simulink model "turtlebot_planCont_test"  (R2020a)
settings: Solver=FixedStepAuto  StartTime=0.0  StopTime=inf  RelTol=1e-3
PreLoadFcn:
  | addpath('../ros_fun')
model workspace (MAT data in the model file):
  SL_ROS_VariableLengthArrays_MaxSizes : object (value not decoded)
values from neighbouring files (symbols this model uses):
  desired_traj = zeros(size(pthObj.States,1),4)    [RRTstar_turtlebot.m]
undefined symbols (not defined in the file or in its folder): nav_msgs, Path, plan
libraries: robotlib x3

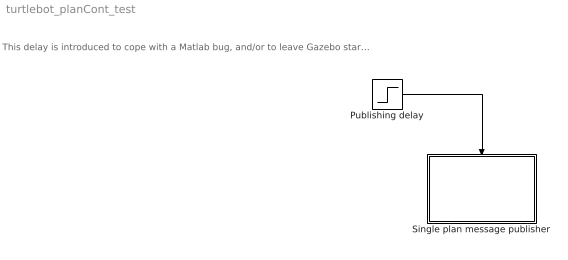
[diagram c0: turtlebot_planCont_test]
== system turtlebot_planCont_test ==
  note: This delay is introduced to cope with a Matlab bug, and/or to leave Gazebo start and initialize correctly before starting the control system
  Publishing delay : Step  Time=5
  Single plan message publisher : Subsystem
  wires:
  Publishing delay/1 -> Single plan message publisher/Enable

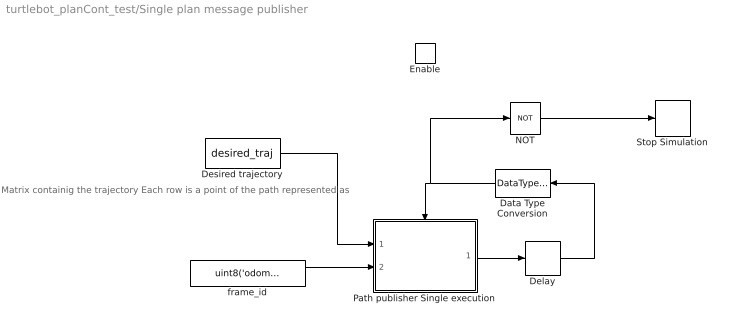
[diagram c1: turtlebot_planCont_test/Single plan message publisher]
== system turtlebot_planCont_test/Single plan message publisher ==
  note: Matrix containig the trajectory Each row is a point of the path represented as
  Enable : EnablePort
  Data Type Conversion : DataTypeConversion  OutDataTypeStr=boolean
  Delay : Delay  InitialCondition=1.0
  Desired trajectory : Constant  Value=desired_traj  VectorParams1D=off
  NOT : Logic  Operator=NOT  IconShape=distinctive  AllPortsSameDT=off  OutDataTypeStr=boolean
  Path publisher Single execution : Subsystem  TreatAsAtomicUnit=on
  Stop Simulation : Stop
  frame_id : Constant  Value=uint8('odom')
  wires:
  NOT/1 -> Stop Simulation/1
  Delay/1 -> Data Type Conversion/1
  frame_id/1 -> Path publisher Single execution/2(frame_id)
  Desired trajectory/1 -> Path publisher Single execution/1(path)
  Path publisher Single execution/1(Enable signal) -> Delay/1
  Data Type Conversion/1 -> NOT/1, Path publisher Single execution/Enable

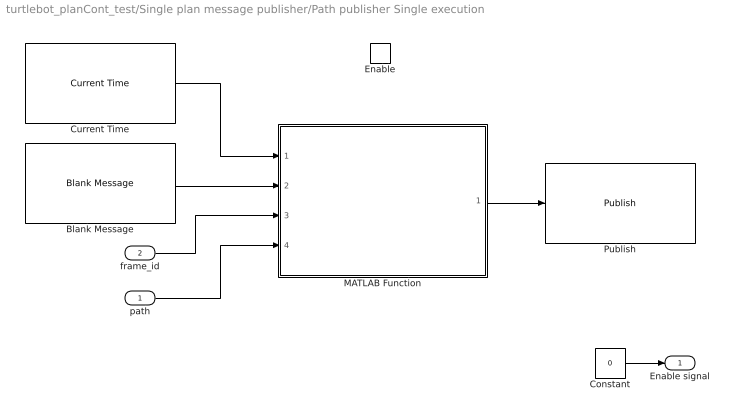
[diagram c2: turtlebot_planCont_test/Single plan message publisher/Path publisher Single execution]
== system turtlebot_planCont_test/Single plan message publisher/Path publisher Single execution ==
  path : Inport
  frame_id : Inport  Port=2
  Enable : EnablePort
  Blank Message : robotlib/Blank Message  messageClass=Message  entityType=nav_msgs/Path  messageType=nav_msgs/Path  SampleTime=inf
  Constant : Constant  Value=0
  Current Time : robotlib/Current Time  OutputFormat=double  SampleTime=-1  ModelName=turtlebot_planCont_test
  MATLAB Function : MATLAB Function  TreatAsAtomicUnit=on
  Publish : robotlib/Publish  topicSource=Specify your own  topic=/plan  messageType=nav_msgs/Path  messageQueueLength=1
  Enable signal : Outport
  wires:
  Current Time/1 -> MATLAB Function/1(time)
  MATLAB Function/1(pathMsg) -> Publish/1
  path/1 -> MATLAB Function/4(path)
  frame_id/1 -> MATLAB Function/3(frame_id)
  Blank Message/1 -> MATLAB Function/2(blankMsg)
  Constant/1 -> Enable signal/1

== matlab function turtlebot_planCont_test/Single plan message publisher/Path publisher
Single execution/MATLAB Function ==
function pathMsg = generate_path_msg(time,blankMsg,frame_id,path)

% Writing the message header
blankMsg.Header.Stamp.Sec = fix(time);
blankMsg.Header.Stamp.Nsec = fix((time-fix(time))*1e9);
blankMsg.Header.FrameId(1:length(frame_id)) = frame_id;
blankMsg.Header.FrameId_SL_Info.CurrentLength = uint32(length(frame_id));

% Set the number of poses
blankMsg.Poses_SL_Info.CurrentLength = uint32(size(path,1));

for seq=1:size(path,1)
    % Writing the header of each pose
    blankMsg.Poses(seq).Header.Stamp.Sec = fix(path(seq,4));
    blankMsg.Poses(seq).Header.Stamp.Nsec = fix((path(seq,4)-fix(path(seq,4)))*1e9);
    blankMsg.Poses(seq).Header.FrameId(1:length(frame_id)) = frame_id;
    blankMsg.Poses(seq).Header.FrameId_SL_Info.CurrentLength = uint32(length(frame_id));

    % Write pose data
    blankMsg.Poses(seq).Pose.Position.X = path(seq,1);
    blankMsg.Poses(seq).Pose.Position.Y = path(seq,2);
    blankMsg.Poses(seq).Pose.Position.Z = 0;
    
    orientation = eul2quat([0, 0, path(seq,3)], 'ZYX');
    blankMsg.Poses(seq).Pose.Orientation.X = orientation(1);
    blankMsg.Poses(seq).Pose.Orientation.Y = orientation(2);
    blankMsg.Poses(seq).Pose.Orientation.Z = orientation(3);
    blankMsg.Poses(seq).Pose.Orientation.W = orientation(4);
end

pathMsg = blankMsg;
